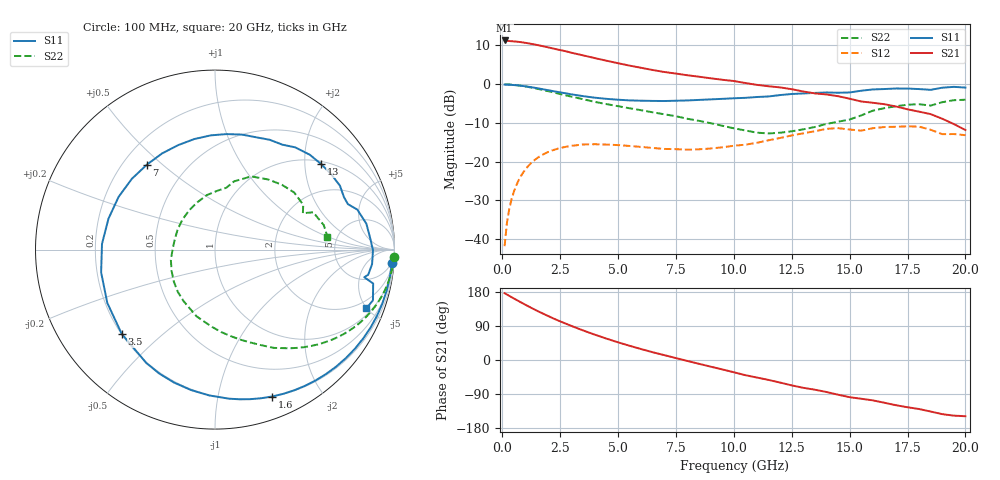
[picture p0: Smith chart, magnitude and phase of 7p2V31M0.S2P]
! Infineon Technologies  Discrete & RF Semiconductors
! bfp620
! VCE =  2.3 V,  IC =  1.0 mA
! Common Emitter S-Parameters:  Sep 2002
# GHz  S  MA  R  50
!  f  S11  S21  S12  S22
! GHz  MAG  ANG  MAG  ANG  MAG  ANG  MAG  ANG
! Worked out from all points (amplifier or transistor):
!   59 points, 100 MHz to 20 GHz, reference 50 ohm
!   highest |S21| = 11.3 dB at 100 MHz (marker M1)
!   |S21| within 3 dB of that: start of sweep to 2.881 GHz
!   unconditionally stable (mu >= 1): 6.289 GHz to 15.72 GHz; 17.95 GHz to 18.91 GHz; 19.63 GHz to end of sweep
!   at 1 GHz: K = 0.10, MSG = 16.3 dB, |S12| = -22.0 dB
!   at 5.5 GHz: K = 0.83, MSG = 10.4 dB, |S12| = -16.0 dB
!   at 20 GHz: K = 1.28, MAG = -2.5 dB, |S12| = -13.2 dB
!   S11 on the Smith chart (normalised r, x): 100 MHz: 4, -26; 1.6 GHz: 0.20, -1.44; 3.5 GHz: 0.20, -0.37; 7 GHz: 0.30, +0.44; 13 GHz: 1.08, +2.42; 20 GHz: 1.38, -4.98
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0.1  0.9883 -4.3  3.672 176.2  0.0081 85.1  0.9982 -2.3
0.2  0.9861 -8.9  3.634 172.8  0.0162 83.7  0.9955 -4.6
0.3  0.9834 -13.4  3.609 169.3  0.0244 81.7  0.9915 -6.9
0.6  0.9694 -26.7  3.548 159.0  0.049 74.1  0.973 -13.5
1.1  0.9292 -48.2  3.382 142.5  0.0864 60.0  0.9237 -23.7
1.6  0.8779 -68.8  3.166 127.0  0.116 46.9  0.8614 -32.8
2  0.8343 -84.6  2.982 115.5  0.1338 37.6  0.8101 -39.1
2.4  0.7937 -99.7  2.802 104.5  0.1472 29.2  0.7599 -44.9
3  0.7386 -121.2  2.543 89.5  0.1602 18.0  0.6893 -52.9
3.5  0.7004 -137.9  2.353 77.8  0.1667 9.9  0.639 -59.0
4  0.6696 -153.7  2.172 66.7  0.1679 2.2  0.5907 -64.3
5  0.6304 177.1  1.866 46.6  0.1636 -8.7  0.5201 -74.5
6  0.6122 151.3  1.628 28.8  0.1549 -16.3  0.461 -85.6
7  0.6066 128.8  1.437 12.8  0.1459 -20.0  0.4086 -97.7
9  0.6369 92.1  1.192 -17.6  0.1478 -21.1  0.3137 -131.3
10.5  0.6668 69.7  1.036 -40.1  0.1657 -23.6  0.2525 -166.8
13  0.7596 38.8  0.805 -73.4  0.2323 -35.7  0.2613 123.7
13.5  0.7717 32.9  0.761 -78.4  0.2471 -40.4  0.2801 111.3
16  0.8556 9.7  0.576 -106.5  0.2702 -64.6  0.455 63.7
17  0.8803 -0.3  0.516 -119.3  0.282 -77.2  0.5191 44.1
18.5  0.8459 -10.5  0.411 -136.0  0.258 -100.5  0.5299 22.5
20  0.9049 -21.2  0.256 -148.4  0.2197 -106.9  0.6304 6.6
